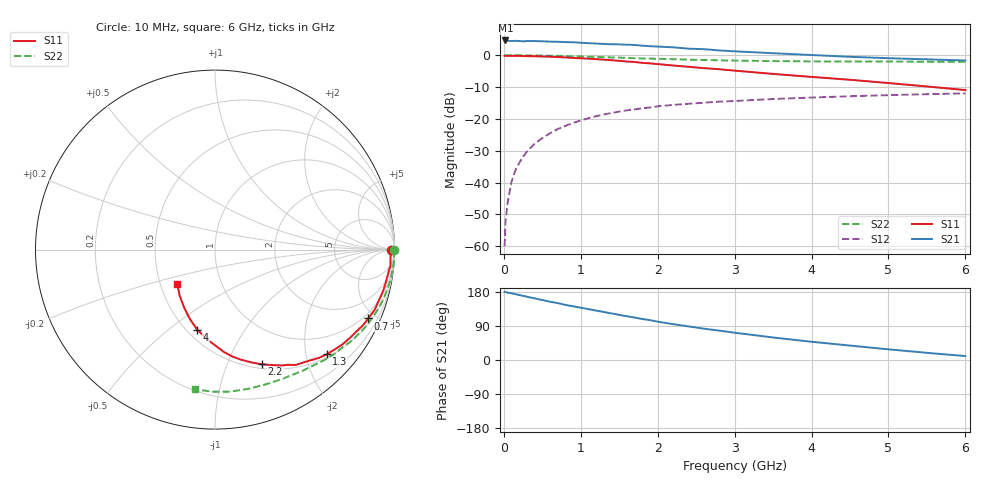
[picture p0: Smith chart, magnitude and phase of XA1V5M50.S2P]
! SIEMENS Discrete & RF Semiconductors
! BFY180
! Si NPN RF Bipolar Junction Transistor in MICRO-X
! VCE = 1.5 V  IC = 0.5 mA
! Common Emitter S-Parameters:  May  1997
# GHz  S  MA  R  50
!  f  S11  S21  S12  S22
! GHz  MAG  ANG  MAG  ANG  MAG  ANG  MAG  ANG
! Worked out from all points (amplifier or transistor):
!   36 points, 10 MHz to 6 GHz, reference 50 ohm
!   highest |S21| = 4.7 dB at 20 MHz (marker M1)
!   |S21| within 3 dB of that: start of sweep to 2.732 GHz
!   unconditionally stable (mu >= 1): 4.887 GHz to end of sweep
!   at 250 MHz: K = 0.05, MSG = 18.1 dB, |S12| = -31.8 dB
!   at 1.4 GHz: K = 0.41, MSG = 10.8 dB, |S12| = -18.1 dB
!   at 6 GHz: K = 1.04, MAG = 4.0 dB, |S12| = -12.0 dB
!   S11 on the Smith chart (normalised r, x): 10 MHz: 96, -8; 700 MHz: 0.73, -4.55; 1.3 GHz: 0.56, -2.42; 2.2 GHz: 0.55, -1.34; 4 GHz: 0.56, -0.63; 6 GHz: 0.61, -0.25
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0.01  0.9796 -0.1  1.667 179.9  0.001 91.9  0.9999 -0.2
0.02  0.9782 -0.6  1.709 179.2  0.0023 88.6  0.9999 -0.5
0.05  0.979 -1.6  1.685 178.1  0.0049 85.6  0.9989 -1.2
0.1  0.9796 -3.6  1.677 176.0  0.0103 88.8  0.9984 -2.4
0.15  0.9822 -5.3  1.687 173.8  0.0156 87.1  0.9993 -3.5
0.2  0.9763 -6.6  1.673 171.4  0.0202 84.9  0.9972 -4.7
0.25  0.9717 -9.0  1.656 169.4  0.0256 84.1  0.9972 -5.9
0.4  0.9646 -13.8  1.673 162.7  0.0408 79.8  0.9933 -9.3
0.6  0.9505 -20.6  1.639 153.7  0.0595 74.2  0.9829 -13.9
0.7  0.9364 -24.2  1.628 150.2  0.0693 71.0  0.9782 -16.2
0.9  0.9087 -30.4  1.602 141.8  0.0865 66.2  0.9642 -20.6
1.1  0.8849 -36.6  1.548 134.2  0.1025 61.4  0.95 -24.8
1.3  0.8536 -43.1  1.506 126.7  0.1175 56.6  0.9342 -28.9
1.7  0.784 -55.1  1.451 112.0  0.1412 48.5  0.898 -36.5
2.2  0.6908 -67.7  1.333 94.6  0.1659 39.6  0.8672 -45.1
2.6  0.6283 -77.0  1.247 82.7  0.1797 34.0  0.8422 -51.1
3  0.5736 -84.9  1.154 72.0  0.1911 28.5  0.8241 -56.9
3.5  0.5092 -93.7  1.077 59.4  0.2053 23.2  0.8105 -63.4
4  0.4571 -102.5  1.009 48.1  0.2166 17.9  0.8014 -70.2
4.5  0.412 -109.8  0.946 38.1  0.227 13.2  0.7972 -77.0
5.5  0.3234 -127.5  0.863 18.9  0.2446 4.0  0.7916 -90.9
6  0.284 -137.9  0.827 10.4  0.2518 -0.8  0.7867 -98.0
